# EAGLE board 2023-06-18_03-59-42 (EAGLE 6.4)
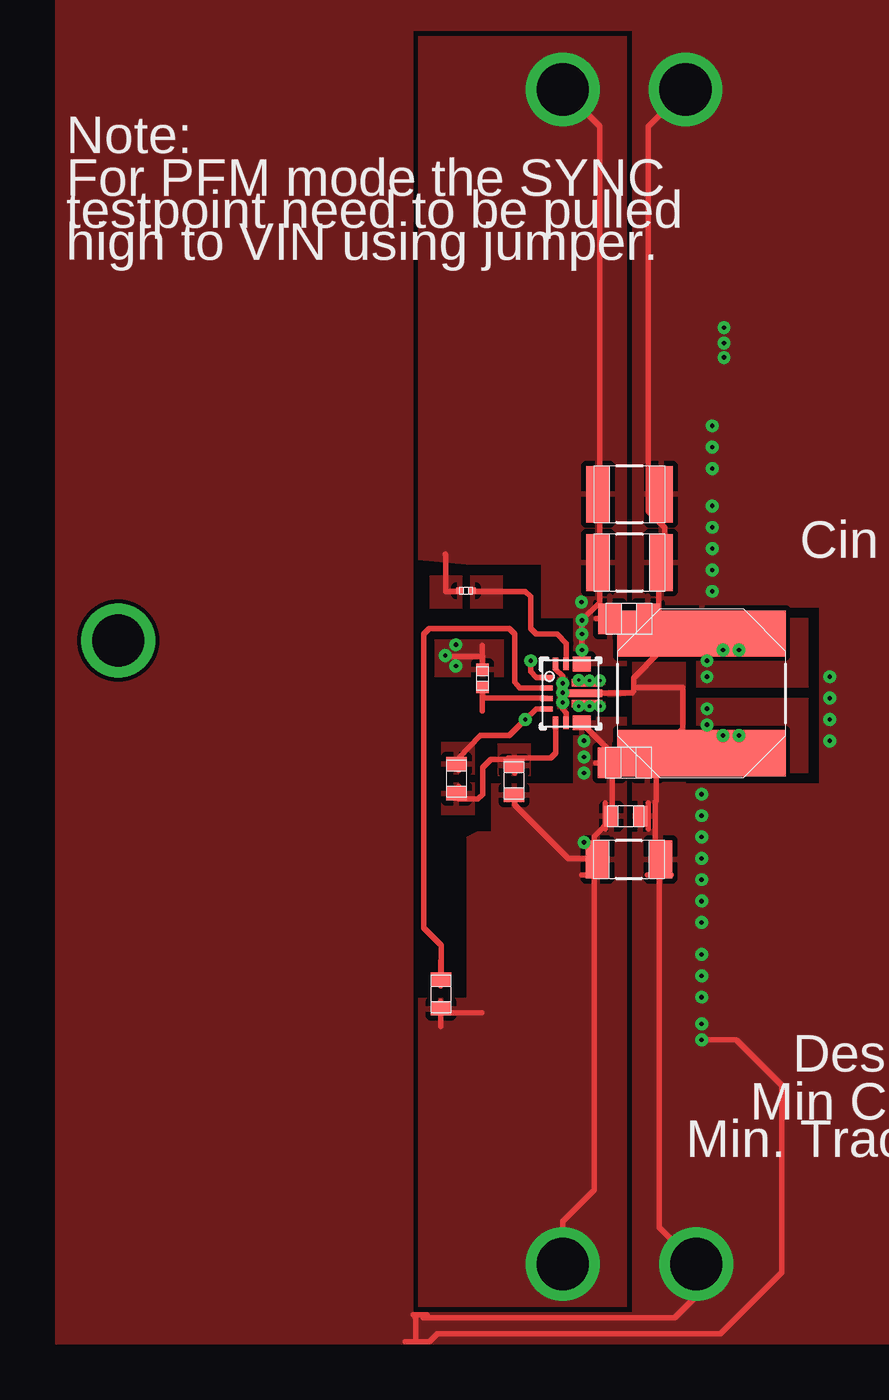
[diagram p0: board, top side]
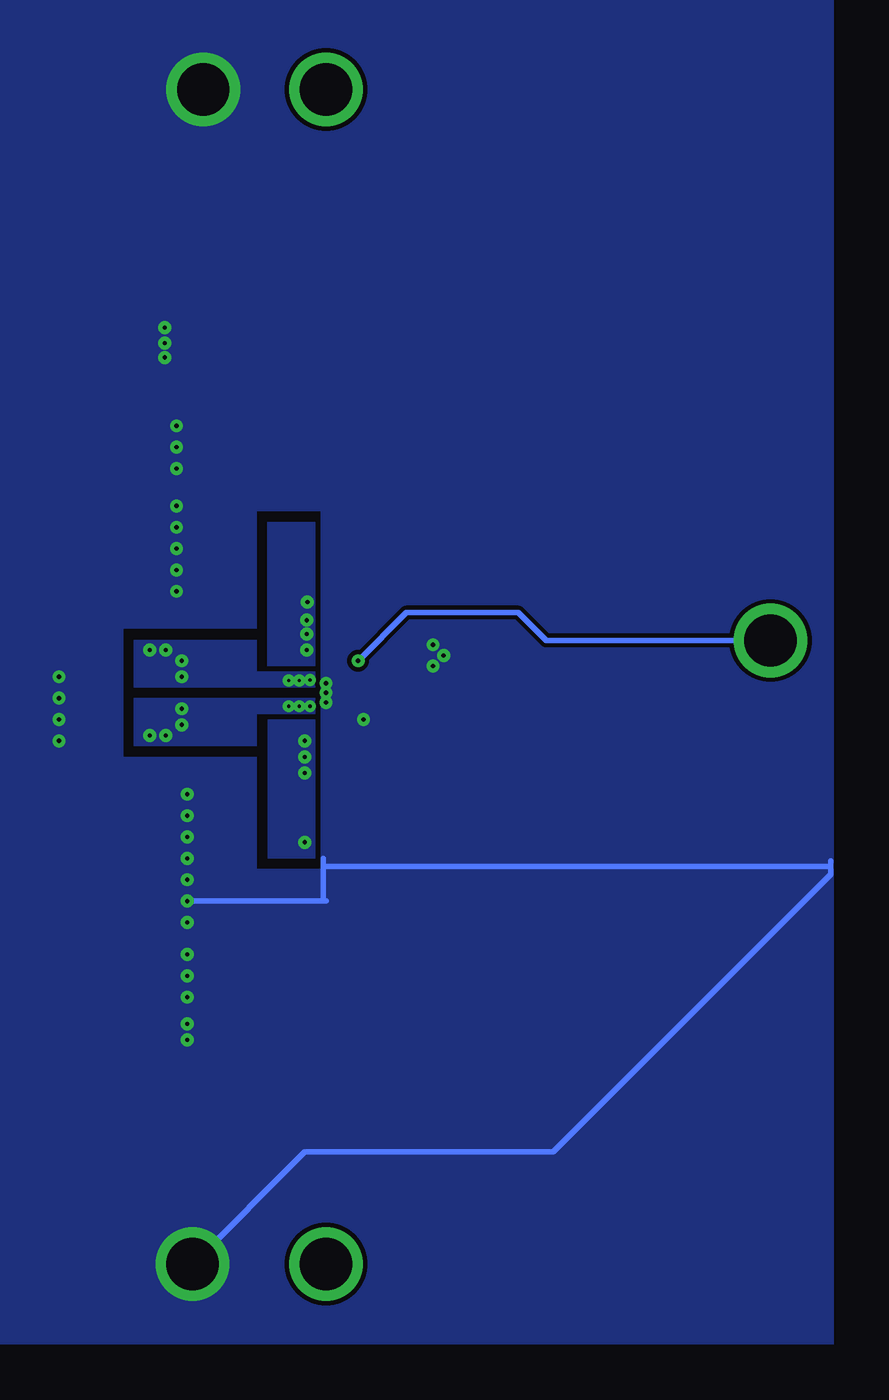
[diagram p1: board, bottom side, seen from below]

No outline drawn. Coordinates in mm, seen from the top.
Copper layers ((1*2)+(15*16)): TOP / INTERNAL1 / layer 15 / BOTTOM

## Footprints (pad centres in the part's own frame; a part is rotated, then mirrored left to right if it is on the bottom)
0805 = smd 1.118 x 1.448: 1 -0.902,0; 2 0.902,0
0402 = smd 0.559 x 0.61: 1 -0.419,0; 2 0.419,0
1210 = smd 1.118 x 2.692: 1 -1.499,0; 2 1.499,0
1206_190 = smd 1.118 x 1.803: 1 -1.499,0; 2 1.499,0
0603 = smd 0.66 x 0.965: 1 -0.699,0; 2 0.699,0
TP-1502 = drill 0.813 pad 1.651 round: 1 0,0
SRN8040 = smd 2.2 x 8: 1 -2.85,0; 2 2.85,0
0201 = smd 0.356 x 0.33: 1 -0.292,0; 2 0.292,0
RNM0015A = smd 0.6 x 0.24: 1 -1.15,0.75; 2 -1.15,0.25; 3 -1.15,-0.25; 4 -1.15,-0.75 | smd 0.24 x 0.6: 5 -0.725,-1.4; 6 -0.225,-1.4; 14 -0.225,1.4; 15 -0.725,1.4 | smd 0.85 x 0.7: 7 0.525,-1.4; 8 0.525,-1.4; 12 0.525,1.4; 13 0.525,1.4 | smd 1.45 x 0.35: 9 0.775,-0.5; 11 0.775,0.5 | smd 1.8 x 0.35: 10 0.6,0

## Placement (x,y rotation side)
C1  [0805]  53.7,60.93 0 top
C2  [0805]  53.67,54.08 0 top
Caux  [0402]  46.74,58.09 90 top
Cin_1  [1210]  53.72,63.6 0 top
Cin_2  [1210]  53.72,66.85 0 top
Cout  [1206_190]  53.7,49.48 0 top
Coutx  [0603]  53.54,51.54 0 top
GND  [TP-1502]  56.36,86.08 270 top
GND1  [TP-1502]  56.87,30.18 270 top
L1  [SRN8040]  57.15,57.38 270 top
Renable  [0201]  45.95,62.26 0 top
Rfbb  [0603]  45.49,53.31 90 top
Rfbt  [0603]  48.23,53.24 90 top
Rpgood  [0603]  44.75,43.08 90 top
SYNC  [TP-1502]  29.36,59.87 270 top
U1  [RNM0015A]  50.93,57.38 0 top
VIN  [TP-1502]  50.55,86.08 270 top
VOUT  [TP-1502]  50.55,30.18 270 top

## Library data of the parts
C1 = ultra-librarian; RefDes: C1; Type: 08051A100CAT2A
C2 = ultra-librarian; RefDes: C2; Type: 08051A100CAT2A
Caux = ultra-librarian; RefDes: Caux; Type: GRM155R71C104KA88D
Cin_1 Cin_2 = ultra-librarian
Cout = ultra-librarian; RefDes: Cout; Type: GRM31CR60J476KE19L
Coutx = ultra-librarian; RefDes: Coutx; Type: GRM188R60J106ME47D
GND = ultra-librarian; RefDes: GND; Type: TP-1502
GND1 = ultra-librarian; RefDes: GND1; Type: TP-1502
L1 = ultra-librarian; RefDes: L1; Type: SRN8040-1R5Y
Renable = ultra-librarian; RefDes: Renable; Type: RC0201FR-0710KL
Rfbb = ultra-librarian; RefDes: Rfbb; Type: RC0603FR-07100KL
Rfbt = ultra-librarian; RefDes: Rfbt; Type: RC0603FR-07309KL
Rpgood = ultra-librarian; RefDes: Rpgood; Type: CRCW0603100KFKEA
SYNC = ultra-librarian; RefDes: SYNC; Type: TP-1502
U1 = ultra-librarian; RefDes: U1; Type: TPS63070RNMR
VIN = ultra-librarian; RefDes: VIN; Type: TP-1502
VOUT = ultra-librarian; RefDes: VOUT; Type: TP-1502

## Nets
0: C1.2 C2.2 Caux.2 Cin_1.2 Cin_2.2 Cout.2 Coutx.2 GND1.1 GND.1 L1.1 L1.2 Rfbb.2 U1.4 U1.6 U1.10 U1.15
3: C1.1 Cin_1.1 Cin_2.1 Renable.1 SYNC.1 U1.1 U1.12 U1.13 VIN.1
8: Rfbb.1 Rfbt.2 U1.5
10: C2.1 Cout.1 Coutx.1 Rfbt.1 Rpgood.1 U1.7 U1.8 VOUT.1
11: Renable.2 U1.14
14: U1.11
15: U1.9
16: Rpgood.2 U1.2
18: Caux.1 U1.3

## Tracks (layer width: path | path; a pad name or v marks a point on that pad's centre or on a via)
0  (via drill 0.2 pad 0.51, 0.2 pad 0.61, 2.49 pad 3.48)
  TOP 0.254: 45.59,53.72 45.59,54.3 46.63,55.37 48.01,55.37 v48.77,56.13 49.28,56.64 49.78,56.64 | 53.92,57.66 53.92,58.12 55.12,59.31 55.12,62.71 55.4,62.99 55.4,65.25 54.61,66.04 54.61,84.33 v56.39,86.11 | 53.92,57.66 53.92,57.48 53.85,57.4 51.54,57.4 v50.55,57.4 | 53.92,57.66 56.26,57.66 56.26,55.68 54.66,54.1 54.66,53.9 54.99,53.59 54.99,52.25 54.94,52.22 54.94,49.71 55.14,49.53 55.14,48.77 55.14,31.98 v56.9,30.23 56.9,28.7 55.88,27.69 44.2,27.69 | v50.55,57.86 50.55,58.19 50.22,58.52 50.22,58.8 | 46.74,59.13 44.98,59.13 v44.96,59.18 | 44.2,27.69 44.07,27.81 43.43,27.81 43.56,27.69 43.56,26.54 | 43.56,26.54 44.2,26.54 44.58,26.92 58.04,26.92 60.96,29.84 60.96,38.73 58.8,40.89 v57.15,40.89 | 43.92,27.69 44.2,27.69 | 43.05,26.54 43.56,26.54 | 50.72,55.98 50.72,56.44 50.55,56.64 v50.55,56.95 | 54.05,54.08 55.24,54.08 | 54.08,60.94 55.27,60.94 | 54.56,48.74 55.7,48.74 | 54.61,50.93 54.61,52.17 | 46.71,58.47 46.71,59.66
  BOTTOM 0.254: 26.54,49.15 50.67,49.15 | 50.67,49.15 50.67,49.53 | 50.67,47.5 50.67,49.15 | v56.9,30.23 51.56,35.56 39.75,35.56 26.54,48.77 26.54,49.4 | 50.55,47.5 v57.15,47.5
  other vias: 63.25,55.12 63.25,57.15 58.22,73.36 58.22,74.78 58.22,74.04 57.15,46.48 57.15,42.93 57.66,65.28 57.66,69.09 57.66,63.25 57.66,70.1 57.66,62.23 57.66,66.29 45.47,58.67 45.47,59.69 63.25,56.13 57.66,64.26 57.66,68.07 57.15,51.56 57.15,52.58 57.15,49.53 57.15,50.55 57.15,48.51 57.15,43.94 57.15,44.96 57.15,41.66 63.25,58.17
  pour TOP (rank 5): 44.78,53.52 44.78,55.07 46.35,55.07 46.35,53.52
  pour TOP (rank 6): 44.45,59.94 44.45,58.17 47.75,58.17 47.75,59.94
  pour TOP (rank 6): 26.42,26.42 26.42,90.42 80.26,90.42 80.26,26.42 53.85,26.42 43.69,26.42 43.69,27.94 53.85,27.94 53.85,56.39 53.85,57.28 50.8,57.02 50.8,56.64 50.29,56.64 50.29,58.17 50.8,58.17 50.8,57.53 56.39,57.53 56.39,53.09 62.74,53.09 62.74,61.47 56.39,61.47 56.39,57.66 53.85,57.66 53.85,88.9 43.43,88.9 43.43,26.42
  pour BOTTOM (rank 6): 80.26,90.42 80.26,26.42 51.56,26.42 26.42,26.42 26.42,49.02 53.85,49.02 53.85,54.36 60.2,54.36 60.2,60.45 53.85,60.45 53.85,66.04 50.8,66.04 50.8,49.28 26.42,49.28 26.42,90.42
3  (via drill 0.2 pad 0.61, 2.49 pad 3.48)
  TOP 0.254: 45.59,62.23 44.98,62.23 44.98,63.96 44.96,64.01 | 51.46,58.8 51.44,58.8 51.46,58.8 | v49.02,58.93 49.02,58.42 49.28,58.14 U1.1 | 51.46,58.8 v51.46,60.86 52.3,61.7 52.3,84.35 v50.55,86.11 | 52.15,60.94 53.34,60.94
  BOTTOM 0.254: v49.02,58.93 46.74,61.21 41.4,61.21 40.08,59.89 v29.41,59.89
  other vias: 51.46,60.2 51.44,61.72 51.46,59.44
  pour TOP: 44.22,61.42 44.22,62.99 45.77,62.99 45.77,61.42
  pour TOP (rank 3): 53.59,58.67 51.05,58.67 51.05,60.96 49.53,60.96 49.53,63.5 45.97,63.5 43.69,63.73 43.69,67.56 43.69,88.65 45.72,88.65 46.3,88.65 50.29,88.65 53.59,88.65
  pour BOTTOM (rank 2): 53.34,58.67 53.34,65.53 51.05,65.53 51.05,58.67
8
  TOP 0.254: 47.95,54.3 48.34,54.3 | 48.26,53.59 48.26,54.23 | 48.34,54.3 49.99,54.3 50.22,54.53 50.22,55.98 | 48.26,54.23 48.34,54.3 | 45.59,52.96 45.59,52.35 46.51,52.35 46.74,52.58 46.74,53.85 47.12,54.23 48.26,54.23
  pour TOP: 44.78,51.59 44.78,53.14 46.35,53.14 46.35,51.59
  pour TOP: 47.45,53.44 47.45,54.99 49.02,54.99 49.02,53.44
10  (via drill 0.2 pad 0.61, 2.49 pad 3.48)
  TOP 0.254: 51.44,55.98 52.91,54.51 52.91,51.46 52.05,50.57 52.05,49.53 | 48.26,52.27 48.26,52.07 50.04,50.29 50.8,49.53 52.05,49.53 | v50.55,30.23 50.55,32.26 52.05,33.76 52.05,49.53 | 44.96,42.19 46.69,42.19 | 52.12,54.08 53.31,54.08 | 51.46,48.74 52.6,48.74 | 52.58,50.93 52.58,52.17 | 44.76,41.53 44.76,42.72
  other vias: 51.56,50.29 51.56,55.12 51.56,54.36 51.56,53.59
  pour TOP (rank 5): 53.59,28.19 53.59,56.26 51.05,56.26 51.05,55.63 51.05,53.59 51.05,53.09 47.14,53.09 47.14,50.8 46.48,50.8 45.97,50.55 45.97,42.9 43.69,42.9 43.69,28.19
  pour BOTTOM (rank 2): 51.05,49.53 53.31,49.53 53.31,56.13 51.05,56.13
11
  TOP 0.254: 46.35,62.23 46.94,62.23 48.77,62.23 49.02,61.98 49.02,60.45 49.28,60.2 50.29,60.2 50.72,59.74 50.72,58.8
  pour TOP (rank 2): 46.15,61.42 46.15,62.99 47.7,62.99 47.7,61.42
14  (via drill 0.15 pad 0.46, 0.2 pad 0.61)
  other vias: 58.17,59.44 57.4,58.17 57.4,58.93 58.93,59.44 52.32,57.99 51.82,57.99 51.31,58.01
  pour TOP (rank 4): 56.9,57.66 56.9,60.96 62.23,60.96 62.23,57.66
  pour TOP (rank 4): 52.58,58.29 52.58,57.78 51.05,57.78 51.05,58.29
  pour BOTTOM (rank 3): 59.69,57.66 51.05,57.66 51.05,58.42 53.85,58.42 53.85,59.92 59.69,59.92
15  (via drill 0.15 pad 0.46, 0.2 pad 0.61)
  other vias: 58.93,55.37 58.17,55.37 57.4,55.88 57.4,56.64 52.32,56.77 51.82,56.77 51.31,56.77
  pour TOP (rank 4): 56.9,57.15 62.23,57.15 62.23,53.59 56.9,53.59
  pour TOP (rank 5): 52.58,56.52 51.05,56.52 51.05,57.02 51.44,57.02 51.82,57.02 52.58,57.02
  pour BOTTOM (rank 3): 51.05,57.15 51.05,56.39 52.88,56.39 53.85,56.39 53.85,54.86 59.69,54.86 59.69,57.15 54.36,57.15
16
  TOP 0.254: 44.78,44.07 44.78,45.39 43.94,46.23 43.94,60.2 44.2,60.45 48.01,60.45 48.26,60.2 48.26,57.91 48.51,57.63 U1.2 | 44.76,43.46 44.76,44.65
18
  TOP 0.254: 46.74,57.17 46.76,57.15 49.78,57.15 | 46.74,57.17 46.74,57.78 | 46.74,57.12 46.74,57.17 | 46.71,56.54 46.71,57.73

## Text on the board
ASSYNOTES: Note: | For PFM mode the SYNC | testpoint need to be pulled | high to VIN using jumper. | Cin | Design Rules: | Min Clearance: 10mil | Min. Track Width : 10 mil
